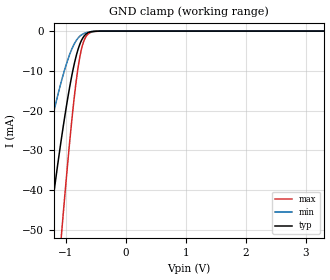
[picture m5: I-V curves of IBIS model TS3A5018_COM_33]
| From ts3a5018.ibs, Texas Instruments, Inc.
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[Model]   TS3A5018_COM_33
Model_type  Terminator
| variable   typ   min   max
C_comp   6.44pF   5.52pF   7.21pF
| C_tri-state   6.44pF   5.52pF   7.21pF
[Temperature Range]   40   100   -40
| Ambient temperature   25   85   -40
[Voltage range]   3.3   3   3.6
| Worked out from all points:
|   GND clamp passes 1 mA (typ) near -0.68 V on its own axis
[GND Clamp]
| TS3A5018_COM_33
|   Voltage   I(typ)   I(min)   I(max)
-3.3V     -396.1mA   -258.1mA   -578.3mA
-1.6V     -93.38mA   -52.07mA   -157.7mA
-1.56V    -87.58mA   -48.45mA   -148.9mA
-1.28V    -50.29mA   -25.82mA   -90.32mA
-1.075V   -27.19mA   -12.69mA   -51.6mA
-955mV    -15.73mA   -6.691mA   -30.97mA
-855mV    -7.986mA   -3.101mA   -16.1mA
-780mV    -3.869mA   -1.478mA   -7.699mA
-710mV    -1.573mA   -693.8uA   -2.954mA
-615mV    -316.5uA   -240.4uA   -579.4uA
-440mV    -10.8uA    -8.179uA   -25.59uA
3.3V      1.763nA    252.3pA    19.12nA
